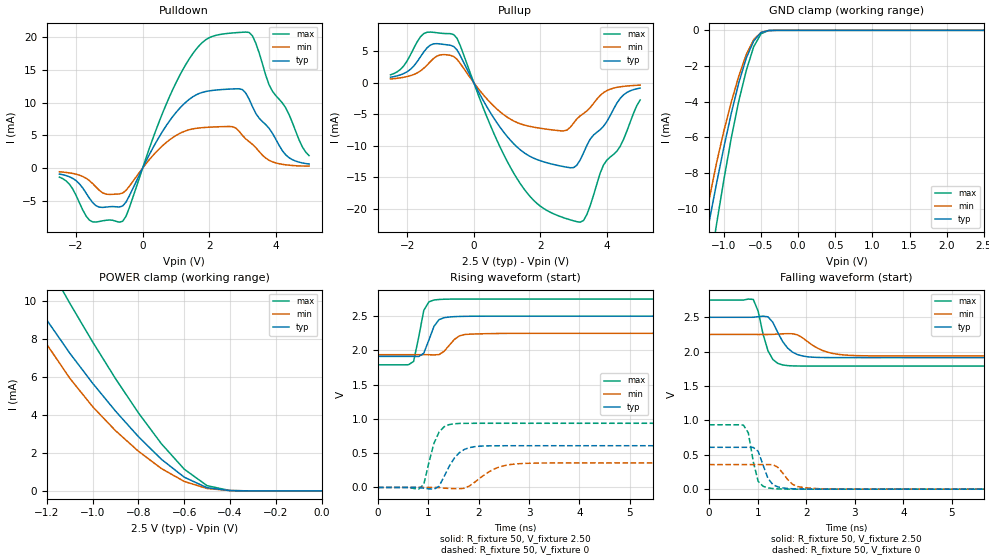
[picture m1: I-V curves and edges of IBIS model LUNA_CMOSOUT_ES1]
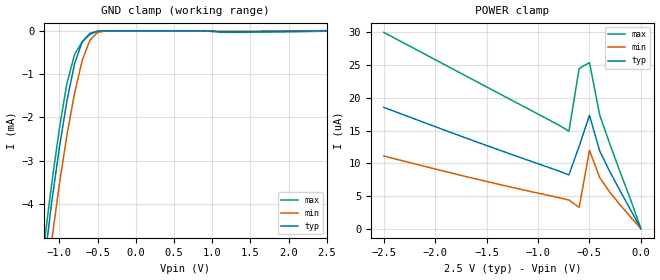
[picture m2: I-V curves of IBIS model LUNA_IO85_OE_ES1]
[IBIS Ver]   3.2
[Comment Char]   |_char
[File name]   sg-9101cga_25v_c.ibs
[File Rev]   1.0
[Date]   2018/09/14 17:36:19
[Source]
[Notes]
[Disclaimer]
This information is for modeling purposes only, and is not guaranteed.
Property of SEIKO EPSON Corp.,
unauthorized reproduction and/or distribution is strictly prohibited.
[Copyright]
Copyright 2018, SEIKO EPSON Corp.
[Component]   SG-9101CGA
Si_location Pin
Timing_location Pin
[Manufacturer]   SEIKO EPSON Corp.
| 2520 PKG
| 2520 PKG
[Package]
R_pkg   238m   NA   NA
L_pkg   2.1n   NA   NA
C_pkg   0.38p   NA   NA
[Pin] signal_name   model_name
1   OE   LUNA_IO85_OE_ES1
2   VSS   GND
3   OUT   LUNA_CMOSOUT_ES1
4   VDD   POWER
| Models and submodels in the file (2): LUNA_CMOSOUT_ES1 (3-state), LUNA_IO85_OE_ES1 (Input)
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[Model]   LUNA_CMOSOUT_ES1
Model_type 3-state
Enable Active-High
Polarity Non-Inverting
Vmeas=1.25
C_comp   2.5p   2.0p   3.0p
[Temperature Range] 25   105   -40
[Voltage Range]   2.50   2.25   2.75
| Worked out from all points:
|   slope of the pulldown table from 0 to 0.375 V, typ, clamps not added: 101 ohm
|   slope of the pullup table from 0 to 0.375 V, typ, clamps not added: 103 ohm
|   GND clamp passes 1 mA (typ) near -0.64 V on its own axis
|   POWER clamp passes 1 mA (typ) near -0.63 V on its own axis
|   falling waveform, R_fixture 50, V_fixture 2.50: 20-80 % time 311ps typ, 456ps min, 218ps max; typ from 2.5 V to 1.91 V
|   falling waveform, R_fixture 50, V_fixture 0: 20-80 % time 209ps typ, 265ps min, 160ps max; typ from 0.609 V to 0 V
|   rising waveform, R_fixture 50, V_fixture 2.50: 20-80 % time 197ps typ, 241ps min, 155ps max; typ from 1.91 V to 2.5 V
|   rising waveform, R_fixture 50, V_fixture 0: 20-80 % time 304ps typ, 455ps min, 221ps max; typ from 0 V to 0.609 V
[Pullup]
-2.5V     844.7uA    573.5uA    1.224mA
-2.1V     1.433mA    839.1uA    2.651mA
-1.5V     4.851mA    2.263mA    7.762mA
-600mV    5.713mA    4.12mA     7.592mA
600mV     -5.599mA   -3.718mA   -7.994mA
1.4V      -10.66mA   -6.539mA   -16.03mA
2.7V      -13.32mA   -7.664mA   -21.42mA
3.2V      -12.25mA   -5.271mA   -22.13mA
3.4V      -9.942mA   -4.492mA   -20.9mA
3.9V      -6.923mA   -1.595mA   -13.06mA
4.4V      -2.504mA   -673.4uA   -10.11mA
5V        -882.1uA   -412.9uA   -2.758mA
[Pulldown]
-2.5V     -901.2uA   -553uA     -1.368mA
-1.6V     -4.583mA   -1.898mA   -7.939mA
-600mV    -5.785mA   -3.808mA   -8.125mA
500mV     4.805mA    2.958mA    7.143mA
1.3V      10.1mA     5.718mA    15.88mA
1.9V      11.73mA    6.235mA    19.65mA
2.7V      12.11mA    6.34mA     20.68mA
3V        12.01mA    5.005mA    20.79mA
3.3V      9.42mA     3.64mA     20.23mA
3.8V      6.085mA    1.202mA    12.73mA
4.3V      2.033mA    511.4uA    9.213mA
5V        637.8uA    321.5uA    1.922mA
[GND Clamp]
-2.5V     -55.19mA   -49.46mA   -64.23mA
-1.3V     -13.11mA   -11.85mA   -16.24mA
-1.2V     -10.77mA   -9.503mA   -13.52mA
-1.1V     -8.591mA   -7.44mA    -10.88mA
-1V       -6.541mA   -5.623mA   -8.358mA
-900mV    -4.635mA   -4.001mA   -6.009mA
-800mV    -2.939mA   -2.563mA   -3.961mA
-700mV    -1.565mA   -1.365mA   -2.263mA
-600mV    -601.2uA   -521.6uA   -925.2uA
-500mV    -121.4uA   -116.4uA   -188.8uA
-300mV    -500.8nA   -1.29uA    -313.5nA
2.5V      140pA      621.1nA    98.8pA
[POWER Clamp]
-2.5V     46.99mA    40.94mA    56.3mA
-1.4V     13.2mA     11.93mA    16.56mA
-1.3V     10.93mA    9.714mA    14.21mA
-1.2V     8.97mA     7.69mA     11.99mA
-1.1V     7.236mA    5.92mA     9.861mA
-1V       5.655mA    4.424mA    7.824mA
-900mV    4.191mA    3.162mA    5.894mA
-700mV    1.665mA    1.179mA    2.483mA
-600mV    721.7uA    498.7uA    1.143mA
-500mV    167.2uA    126.9uA    275.1uA
-400mV    16.41uA    18.75uA    19.76uA
0V        140pA      780.7pA    121.2pA
[Falling Waveform]
R_fixture=50
V_fixture=2.50
V_fixture_min=2.25
V_fixture_max=2.75
0s        2.5V       2.25V      2.75V
909.1ps   2.5V       2.25V      2.76V
1.01ns    2.509V     2.25V      2.589V
1.212ns   2.507V     2.25V      2.014V
1.414ns   2.279V     2.256V     1.83V
1.616ns   2.053V     2.262V     1.797V
2.02ns    1.926V     2.15V      1.79V
2.424ns   1.914V     1.996V     1.79V
2.929ns   1.913V     1.945V     1.79V
10ns      1.913V     1.938V     1.79V
[Falling Waveform]
R_fixture=50
V_fixture=0
V_fixture_min=0
V_fixture_max=0
0s        609mV      357.7mV    936.6mV
707.1ps   609mV      357.7mV    931.3mV
808.1ps   609mV      357.7mV    818.2mV
909.1ps   607.5mV    357.7mV    401.9mV
1.01ns    550mV      357.7mV    114.3mV
1.212ns   156.6mV    358.1mV    18.39mV
1.313ns   66.25mV    356mV      8.816mV
1.717ns   5.981mV    71.97mV    472.9uV
2.121ns   759.7uV    12.53mV    19.71uV
10ns      0V         0V         0V
[Rising Waveform]
R_fixture=50
V_fixture=2.50
V_fixture_min=2.25
V_fixture_max=2.75
0s        1.913V     1.938V     1.79V
606.1ps   1.913V     1.938V     1.791V
707.1ps   1.913V     1.938V     1.84V
909.1ps   1.959V     1.938V     2.584V
1.01ns    2.151V     1.938V     2.709V
1.111ns   2.351V     1.935V     2.736V
1.313ns   2.478V     1.988V     2.748V
1.616ns   2.496V     2.213V     2.75V
1.818ns   2.499V     2.237V     2.75V
10ns      2.5V       2.25V      2.75V
[Rising Waveform]
R_fixture=50
V_fixture=0
V_fixture_min=0
V_fixture_max=0
0s        0V         0V         0V
808.1ps   216.4uV    3.153uV    -24.99mV
909.1ps   -11.49mV   -12.5uV    44.57mV
1.111ns   -25.14mV   533.3uV    644.5mV
1.212ns   16.82mV    -3.048mV   808mV
1.515ns   427.7mV    -16.95mV   929.8mV
1.818ns   581.9mV    22.54mV    936.3mV
2.323ns   608.4mV    274.4mV    936.6mV
2.828ns   609mV      347.8mV    936.6mV
10ns      609mV      357.7mV    936.6mV
[Ramp]
R_load=50
dV/dt_r   3.654E-1/2.981E-10   2.146E-1/4.506E-10   5.620E-1/2.175E-10
dV/dt_f   3.522E-1/3.083E-10   1.874E-1/4.528E-10   5.760E-1/2.160E-10
|[End   LUNA_CMOSOUT_ES1
[Model]   LUNA_IO85_OE_ES1
Model_type Input
Enable Active-Low
Polarity Non-Inverting
Vinh=1.93
Vinl=0.67
C_comp   2.5p   2.0p   3.0p
[Temperature Range] 25   105   -40
[Voltage Range]   2.50   2.25   2.75
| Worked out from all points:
|   GND clamp passes 1 mA (typ) near -0.83 V on its own axis
[GND Clamp]
-2.5V     -32.2mA    -31.31mA   -34.3mA
-1.2V     -5.408mA   -6.351mA   -4.953mA
-1.1V     -3.959mA   -4.854mA   -3.533mA
-1V       -2.702mA   -3.543mA   -2.264mA
-900mV    -1.611mA   -2.406mA   -1.207mA
-800mV    -755.7uA   -1.435mA   -544uA
-700mV    -251.7uA   -679.9uA   -254uA
-600mV    -60.42uA   -218.4uA   -84.78uA
-500mV    -8.306uA   -39.73uA   -10.67uA
-400mV    -801.3nA   -4.121uA   -821nA
1.2V      -21.43uA   -11.22uA   -36.93uA
2.5V      102pA      4.547uA    -9.898uA
[POWER Clamp]
-2.5V     18.55uA    11.12uA    30.01uA
-1.6V     13.28uA    7.586uA    22.5uA
-900mV    9.38uA     5.089uA    16.69uA
-700mV    8.214uA    4.376uA    14.9uA
-600mV    12.61uA    3.264uA    24.49uA
-500mV    17.33uA    11.98uA    25.38uA
-400mV    11.86uA    7.796uA    17.35uA
-300mV    8.666uA    5.523uA    12.86uA
-100mV    2.864uA    1.778uA    4.438uA
0V        101.8pA    233pA      102.9pA
